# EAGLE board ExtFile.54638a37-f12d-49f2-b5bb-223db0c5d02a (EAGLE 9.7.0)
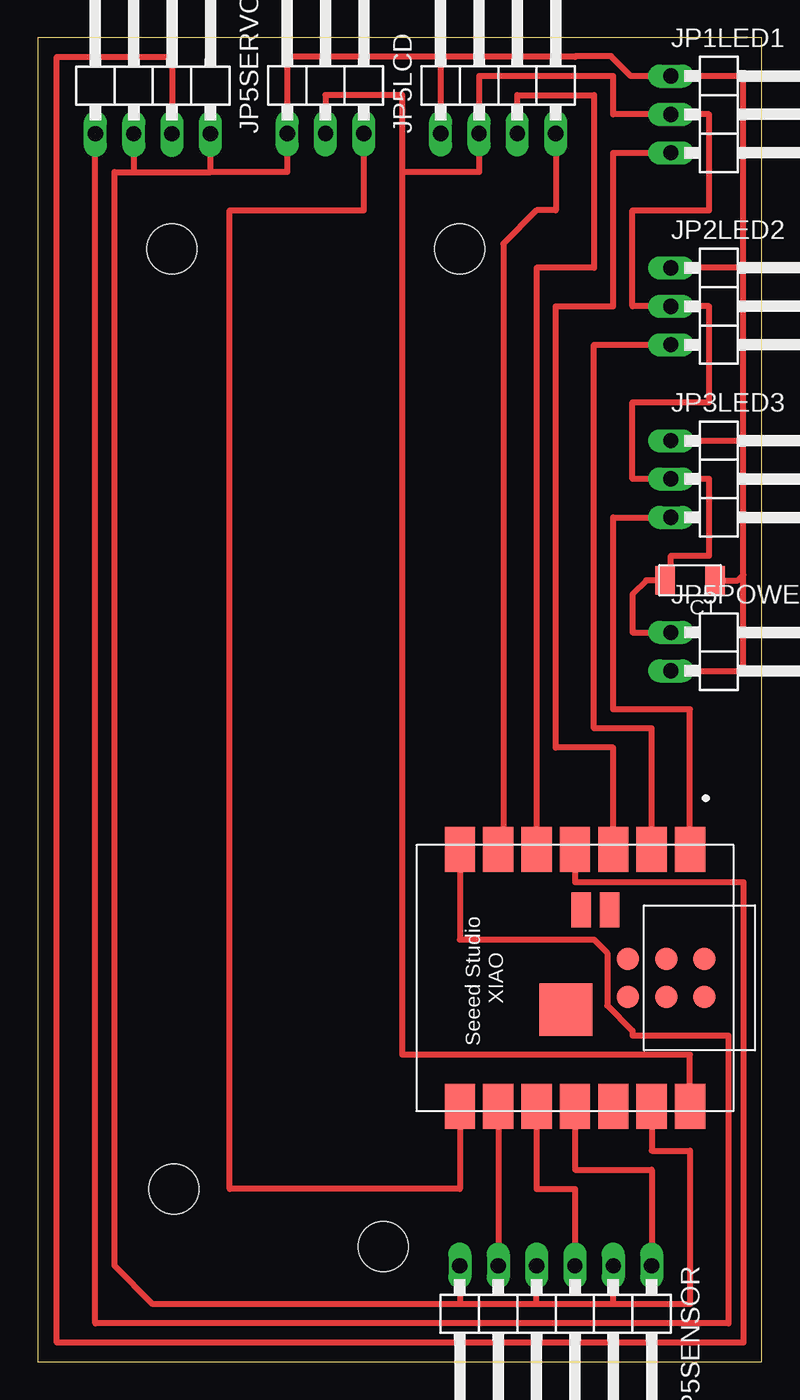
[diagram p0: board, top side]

Size 47.93 x 87.62 mm. Coordinates in mm from the lower left corner, seen from the top.
Outline: 0,0 47.93,0 47.93,87.62 0,87.62 0,0
Copper layers (1*16): Top / Bottom
Stack-up Default Layer Stack: Top User Defined 0.035mm / Dielectric-1 User Defined 1.5mm / Bottom User Defined 0.035mm
Design rules: minimum copper width 10mil, minimum drill size 32mil, copper clearance wire_polygon to wire_polygon 16mil, copper clearance wire_polygon to pad_smd 16mil, copper clearance wire_polygon to via 16mil, copper clearance pad_smd to pad_smd 16mil, copper clearance pad_smd to via 16mil, copper clearance via to via 16mil, copper clearance smd to pad (same net) 16mil, copper clearance smd to via (same net) 16mil, copper clearance smd to smd (same net) 16mil, dimension clearance 40mil, via restrict clearance 0mil, restrict clearance 0mil, drill distance 16mil, keepout clearance 0mil
Holes 3.3 mm at 27.94,73.66 8.89,73.66 9.02,11.43 22.86,7.62

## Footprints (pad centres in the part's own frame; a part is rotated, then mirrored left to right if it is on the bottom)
C1206FAB = smd 1.27 x 1.905: 1 -1.651,0; 2 1.651,0
1X03/90 = drill 1.016 long: 1 -2.54,-3.81; 2 0,-3.81; 3 2.54,-3.81
1X04/90 = drill 1.016 long: 1 -3.81,-3.81; 2 -1.27,-3.81; 3 1.27,-3.81; 4 3.81,-3.81
1X02/90 = drill 1.016 long: 1 -1.27,-3.81; 2 1.27,-3.81
1X06/90 = drill 1.016 long: 1 -6.35,-3.81; 2 -3.81,-3.81; 3 -1.27,-3.81; 4 1.27,-3.81; 5 3.81,-3.81; 6 6.35,-3.81
XIAO-ESP32C3-MODULE14P-2.54-21X17.8MM = smd 3 x 2: 1 -8.5,7.62; 2 -8.5,5.08; 3 -8.5,2.54; 4 -8.5,0; 5 -8.5,-2.54; 6 -8.5,-5.08; 7 -8.5,-7.62; 8 8.5,-7.62; 9 8.5,-5.08; 10 8.5,-2.54; 11 8.5,0; 12 8.5,2.54; 13 8.5,5.08; 14 8.5,7.62 | smd 1.5 x 1.5: 15 -1.27,8.58; 16 1.27,8.58; 17 -1.27,6.04; 18 1.27,6.04; 19 -1.27,3.5; 20 1.27,3.5 | smd 2.3 x 1.3: 21 -4.5,2.3; 22 -4.5,0.4 | smd 3.5 x 3.5: 23 2.1,-0.6

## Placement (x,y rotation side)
C1  [C1206FAB]  43.18,51.71 180 top
JP1LED1  PINHD-1X3/90  [1X03/90]  45.72,82.55 270 top
JP2LED2  PINHD-1X3/90  [1X03/90]  45.72,69.85 270 top
JP3LED3  PINHD-1X3/90  [1X03/90]  45.72,58.42 270 top
JP5BTN  PINHD-1X4/90  [1X04/90]  7.62,85.08 0 top
JP5LCD  PINHD-1X4/90  [1X04/90]  30.48,85.09 0 top
JP5POWERGND  PINHD-1X2/90  [1X02/90]  45.72,46.99 270 top
JP5SENSOR  PINHD-1X6/90  [1X06/90]  34.29,2.54 180 top
JP5SERVO  PINHD-1X3/90  [1X03/90]  19.05,85.09 0 top
U1  XIAO-ESP32C3  [XIAO-ESP32C3-MODULE14P-2.54-21X17.8MM]  35.56,25.4 270 top

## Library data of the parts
C1 = fab
JP1LED1 JP2LED2 JP3LED3 JP5SERVO = Connector; CATEGORY: Headers; DESCRIPTION: Header, Right Angle, 3 Position; MANUFACTURER: Generic; MPN: Generic; OPERATING_TEMPERATURE: Generic; PART_STATUS: Active; PITCH: 0.100" (2.54mm); ROHS_COMPLIANCE: Generic; SERIES: Generic; SUB-CATEGORY: Headers, Male Pins; TYPE: Board to Board or Cable, Unshrouded, Through Hole, Right Angle
JP5BTN JP5LCD = Connector; CATEGORY: Headers; DESCRIPTION: Header, Right Angle, 4 Position; MANUFACTURER: Generic; MPN: Generic; OPERATING_TEMPERATURE: Generic; PART_STATUS: Active; PITCH: 0.100" (2.54mm); ROHS_COMPLIANCE: Generic; SERIES: Generic; SUB-CATEGORY: Headers, Male Pins; TYPE: Board to Board or Cable, Unshrouded, Through Hole, Right Angle
JP5POWERGND = Connector; CATEGORY: Headers; DESCRIPTION: Header, Right Angle, 2 Position; MANUFACTURER: Generic; MPN: Generic; OPERATING_TEMPERATURE: Generic; PART_STATUS: Active; PITCH: 0.100" (2.54mm); ROHS_COMPLIANCE: Generic; SERIES: Generic; SUB-CATEGORY: Headers, Male Pins; TYPE: Board to Board or Cable, Unshrouded, Through Hole, Right Angle
JP5SENSOR = Connector; CATEGORY: CONNECTOR; SUB-CATEGORY: PIN-HEADER
U1 = Seeed Studio XIAO Series

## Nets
BTN1: JP5BTN.3 U1.4
BTN2: JP5BTN.1 U1.7
GND: C1.1 JP1LED1.1 JP2LED2.1 JP3LED3.1 JP5BTN.2 JP5BTN.4 JP5LCD.1 JP5POWERGND.2 JP5SENSOR.2 JP5SENSOR.4 JP5SENSOR.6 JP5SERVO.1 U1.13
INPUT1: JP5SENSOR.1 U1.11
INPUT2: JP5SENSOR.3 U1.10
INPUT3: JP5SENSOR.5 U1.9
LED1: JP3LED3.3 U1.1
LED2: JP2LED2.3 U1.2
LED3: JP1LED1.3 U1.3
SCL: JP5LCD.4 U1.6
SDA: JP5LCD.3 U1.5
SERVO: JP5SERVO.3 U1.8
VCC: C1.2 JP1LED1.2 JP2LED2.2 JP3LED3.2 JP5LCD.2 JP5POWERGND.1 JP5SERVO.2 U1.14

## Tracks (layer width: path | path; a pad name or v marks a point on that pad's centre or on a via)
BTN1
  Top 0.406: U1.4 35.56,31.75 46.71,31.75 46.71,1.27 1.27,1.27 1.27,86.36 8.89,86.36 JP5BTN.3
BTN2  (1 unrouted)
  Top 0.406: U1.7 27.94,27.94 36.83,27.94 37.7,27.07 37.7,23.57 39.37,21.9 39.37,21.59 45.72,21.59 45.72,2.54 3.81,2.54 JP5BTN.1
GND
  Top 0.406: U1.13 40.64,13.97 43.18,13.97 43.18,3.81 38.1,3.81 | 38.1,3.81 JP5SENSOR.2 | 38.1,3.81 33.02,3.81 | 33.02,3.81 JP5SENSOR.4 | 33.02,3.81 27.94,3.81 | JP5SENSOR.6 27.94,3.81 | JP5POWERGND.2 46.71,45.72 46.71,52.07 | 46.71,52.07 46.71,60.96 | 46.71,60.96 46.71,72.39 | 46.71,72.39 JP2LED2.1 | JP3LED3.1 46.71,60.96 | 46.71,72.39 46.71,85.09 JP1LED1.1 39.25,85.09 37.94,86.4 35.6,86.4 35.56,86.36 26.67,86.36 | C1.1 46.36,51.71 46.71,52.07 | 26.67,86.36 16.51,86.36 JP5SERVO.1 16.51,78.74 11.43,78.74 | 26.67,86.36 JP5LCD.1 | 11.43,78.74 JP5BTN.4 | JP5BTN.2 6.35,78.74 | 6.35,78.74 11.43,78.74 | 27.94,3.81 7.62,3.81 5.08,6.35 5.08,78.74 6.35,78.74
INPUT1
  Top 0.406: U1.11 35.56,12.7 40.64,12.7 JP5SENSOR.1
INPUT2
  Top 0.406: U1.10 33.02,11.43 35.56,11.43 JP5SENSOR.3
INPUT3
  Top 0.406: U1.9 JP5SENSOR.5
LED1
  Top 0.406: U1.1 43.18,43.18 38.1,43.18 38.1,55.88 JP3LED3.3
LED2
  Top 0.406: U1.2 40.64,41.91 36.83,41.91 36.83,67.31 JP2LED2.3
LED3
  Top 0.406: U1.3 38.1,40.64 34.29,40.64 34.29,69.85 38.1,69.85 38.1,80.01 JP1LED1.3
SCL
  Top 0.406: U1.6 30.81,34.23 30.81,73.99 33.02,76.2 34.29,76.2 JP5LCD.4
SDA
  Top 0.406: JP5LCD.3 31.75,83.82 36.83,83.82 36.83,72.39 33.02,72.39 U1.5
SERVO
  Top 0.406: U1.8 27.94,11.43 12.7,11.43 12.7,76.2 21.59,76.2 JP5SERVO.3
VCC
  Top 0.406: JP5POWERGND.1 39.37,48.26 39.37,50.8 40.28,51.71 C1.2 41.91,52.09 41.91,53.34 44.45,53.34 44.45,58.42 JP3LED3.2 39.37,58.42 39.37,63.5 44.45,63.5 44.45,69.85 JP2LED2.2 39.37,69.85 39.37,76.2 44.45,76.2 44.45,82.55 JP1LED1.2 38.1,82.55 38.1,85.09 29.21,85.09 JP5LCD.2 29.21,78.74 24.13,78.74 | 24.13,78.74 24.13,83.82 19.05,83.82 JP5SERVO.2 | U1.14 43.18,20.32 24.13,20.32 24.13,78.74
